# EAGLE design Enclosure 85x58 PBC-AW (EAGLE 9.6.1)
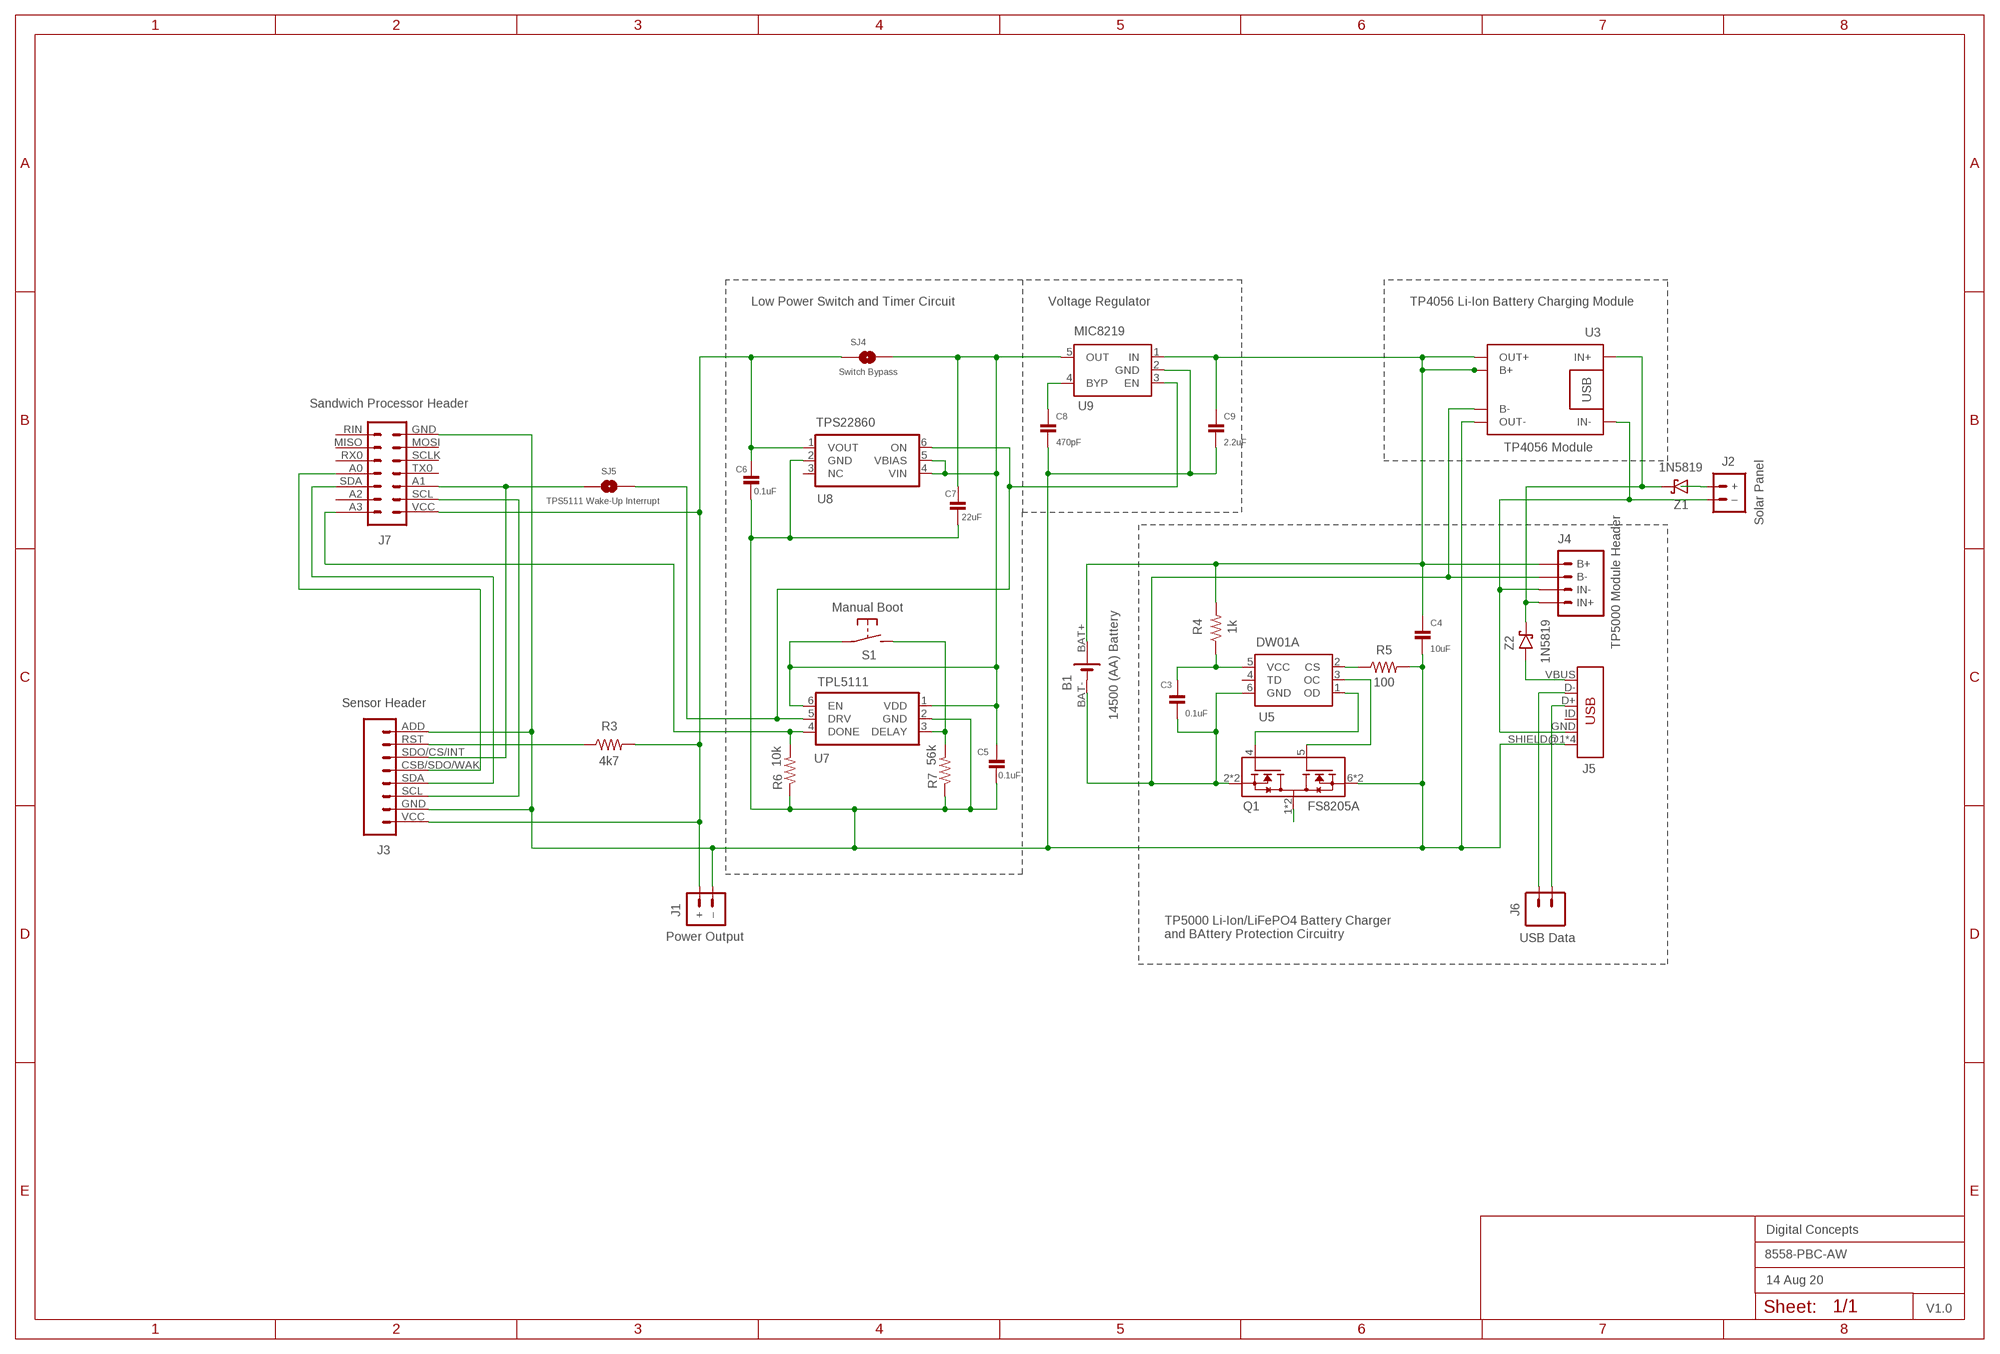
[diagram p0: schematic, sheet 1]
FRAME2 (A3L-LOC): DATE: 14 Aug 20; OWNER: Digital Concepts; TITLE: 8558-PBC-AW; VERSION: V1.0

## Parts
B1  14500 (AA) Battery  BATTERY-HOLDER-14500(AA)  [BATTERY-14500]
C3  0.1uF  CAPACITOR  [C0805]
C4  10uF  CAPACITOR  [C0805]
C5  0.1uF  CAPACITOR  [C0805]
C6  0.1uF  CAPACITOR  [C0805]
C7  22uF  CAPACITOR  [C0805]
C8  470pF  CAPACITOR  [C0805]
C9  2.2uF  CAPACITOR  [C0805]
J1  Power Output  JST-PH1.25-MALE  [JST-PH1.25]
J2  Solar Panel  JST-PH2.0-MALE  [JST-PH2.0]
J3  Sensor Header  HEADER-1X8-SENSOR  [CONN_08-SENSOR]
J4  TP5000 Module Header  TP5000-MODULE  [CONN_04-GENERIC]
J5  USB  USB_MINI-B_SMT  [USB-MINIB]
J6  USB Data  1X2-PIN-HEADER  [CONN_02-GENERIC]
J7  Sandwich Processor Header  HEADER-2X7-SANDWICH-PROCESSOR  [CONN_2X7-WIJNAND-PROCESSOR]
Q1  FS8205A  [SOP65P640X120-8N]
R3  4k7  RESISTORR0805  [R0805]
R4  1k  RESISTORR0805  [R0805]
R5  100  RESISTORR0805  [R0805]
R6  10k  RESISTORR0805  [R0805]
R7  56k  RESISTORR0805  [R0805]
S1  Manual Boot  MOMENTARY-SWITCH-2-PIN  [SWITCH-2-PAD]
SJ4  Switch Bypass  SJ  [SJ]
SJ5  TPS5111 Wake-Up Interrupt  SJ  [SJ]
U3  TP4056 Module  BATTERY-CHARGER-LI-PROT  [BATTERY-CHARGER-LI-PROT]
U5  DW01A  [SOT23-6]
U7  TPL5111  TPL5111DDCR  [SOT-23-6]
U8  TPS22860  [SOT-23-6]
U9  MIC8219  MIC5219XX  [SOT-23-5]
Z1  1N5819  1N5819-SOD-123  [SOD-123]
Z2  1N5819  1N5819-SOD-123  [SOD-123]

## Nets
GND: C4.2 C5.2 C6.2 C7.2 C8.2 C9.2 J1.-(–) J3.ADD J3.GND J5.SHIELD@1(SHIELD) J5.SHIELD@2(SHIELD) J5.SHIELD@3(SHIELD) J5.SHIELD@4(SHIELD) J7.GND Q1.6(S2) Q1.7(S2) R5.2 R6.1 R7.1 U3.OUT- U7.2(GND) U8.2(GND) U9.2(GND)
N$1: J2.+ Z1.A
N$2: J2.-(–) J4.2(IN-) J5.GND U3.IN-
N$3: R5.1 U5.2(CS)
N$4: Q1.1(D12) Q1.8(D12)
N$5: J4.1(IN+) U3.IN+ Z1.C Z2.C
N$6: B1.BAT+ C4.1 C9.1 J4.4(B+) R4.2 U3.B+ U3.OUT+ U9.1(IN)
N$7: C8.1 U9.4(BYP)
N$8: J3.SCL J7.SCL
N$9: J3.RST R3.1
N$10: J3.CSB/SDO/WAK J7.A0
N$11: J3.SDA J7.SDA
N$18: Q1.5(G2) U5.3(OC)
N$19: J5.VBUS Z2.A
N$20: Q1.4(G1) U5.1(OD)
N$21: J5.D+ J6.2
N$22: C3.1 R4.1 U5.5(VCC)
N$23: B1.BAT- C3.2 J4.3(B-) Q1.2(S1) Q1.3(S1) U3.B- U5.6(GND)
N$24: J5.D- J6.1
N$25: R7.2 S1.P$2(S) U7.3(DELAY)
N$26: C5.1 C7.1 S1.P$1(P) SJ4.2 U7.1(VDD) U7.6(EN) U8.4(VIN) U8.5(VBIAS) U9.5(OUT)
N$28: SJ5.2 U7.5(DRV) U8.6(ON) U9.3(EN)
N$29: J7.A3 R6.2 U7.4(DONE)
N$30: J3.SDO/CS/INT J7.A1 SJ5.1
VCC: C6.1 J1.+ J3.VCC J7.VCC R3.2 SJ4.1 U8.1(VOUT)
Unconnected: J5.ID J7.A2 J7.MISO J7.MOSI J7.RIN J7.RX0 J7.SCLK J7.TX0 U5.4(TD) U8.3(NC)

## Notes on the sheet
- Low Power Switch and Timer Circuit | Voltage Regulator | TP4056 Li-Ion Battery Charging Module
- TP5000 Li-Ion/LiFePO4 Battery Charger
  and BAttery Protection Circuitry

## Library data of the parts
B1 = digitalconcepts:BATTERY-HOLDER-14500(AA): 14500 (AA) battery holder
C3-C9 = digitalconcepts:CAPACITOR: 0805 Capacitor
J1 = digitalconcepts:JST-PH1.25-MALE: PH1.25 Male PCB Connector
J2 = digitalconcepts:JST-PH2.0-MALE: PH2.0 Male PCB Connector
J3 = digitalconcepts:HEADER-1X8-SENSOR: IoT Sensors 1x8 Pin Header for 'Sandwich' IoT Sensors
J4 = digitalconcepts:TP5000-MODULE: TP5000 Module Pin Header
J5 = digitalconcepts:USB_MINI-B: USB Mini-B Connector Breaks out 5 pins, and includes shield pins if needed.
J6 = digitalconcepts:1X2-PIN-HEADER: Single Row 2-Pin Header
J7 = digitalconcepts:HEADER-2X7-SANDWICH-PROCESSOR: 'Sandwixh' Processor 2x7 Pin Header for 'Sandwich' Processor/RFM95W PCBs
Q1 = FS8205A:FS8205A: N/A; AVAILABILITY: Unavailable; MF: Fortune Semiconductor; MP: FS8205A; PACKAGE: Package; PRICE: None
R3-R7 = digitalconcepts:RESISTOR: RESISTOR, American symbol; SPICEPREFIX: R
S1 = digitalconcepts:MOMENTARY-SWITCH-2-PIN: 2 Pin Momentary Switch
SJ4 SJ5 = digitalconcepts:SJ: Solder Jumper
U3 = digitalconcepts:BATTERY-CHARGER-LI-PROT: TP4056 Li Battery Charger module with PCB (rather than module) footprint
U5 = DW01A:DW01A; AVAILABILITY: Unavailable; DESCRIPTION: One Cell Lithium-ion/Polymer Battery Protection IC; MF: Fortune Semiconductor; MP: DW01A; PACKAGE: SOT-23-6 Fortune Semiconductor; PRICE: None
U7 = TPL5111DDCR:TPL5111DDCR: TPL5111 Nano-Power System Timer
U8 = TPL5111DDCR:TPS22860: Texas Instruments TPS22860 Ultra-Low Leakage Load Switch
U9 = digitalconcepts:MIC5219XX: VOLTAGE REGULATOR; OC_FARNELL: unknown; OC_NEWARK: unknown
Z1 Z2 = digitalconcepts:1N5819-SOD-123: 1N5819 Schottky Diode SOD-123

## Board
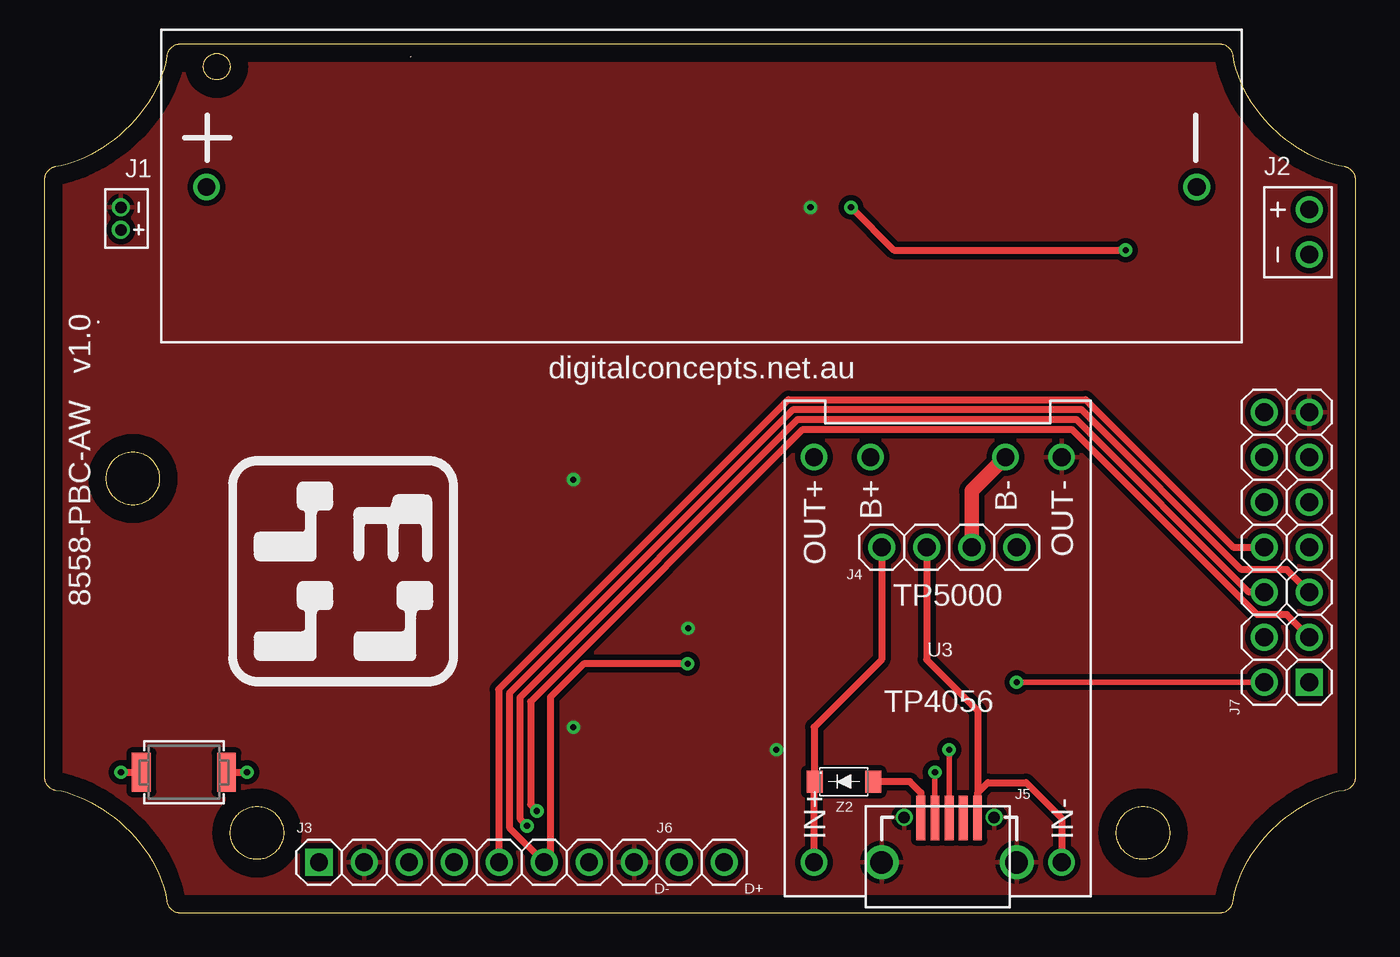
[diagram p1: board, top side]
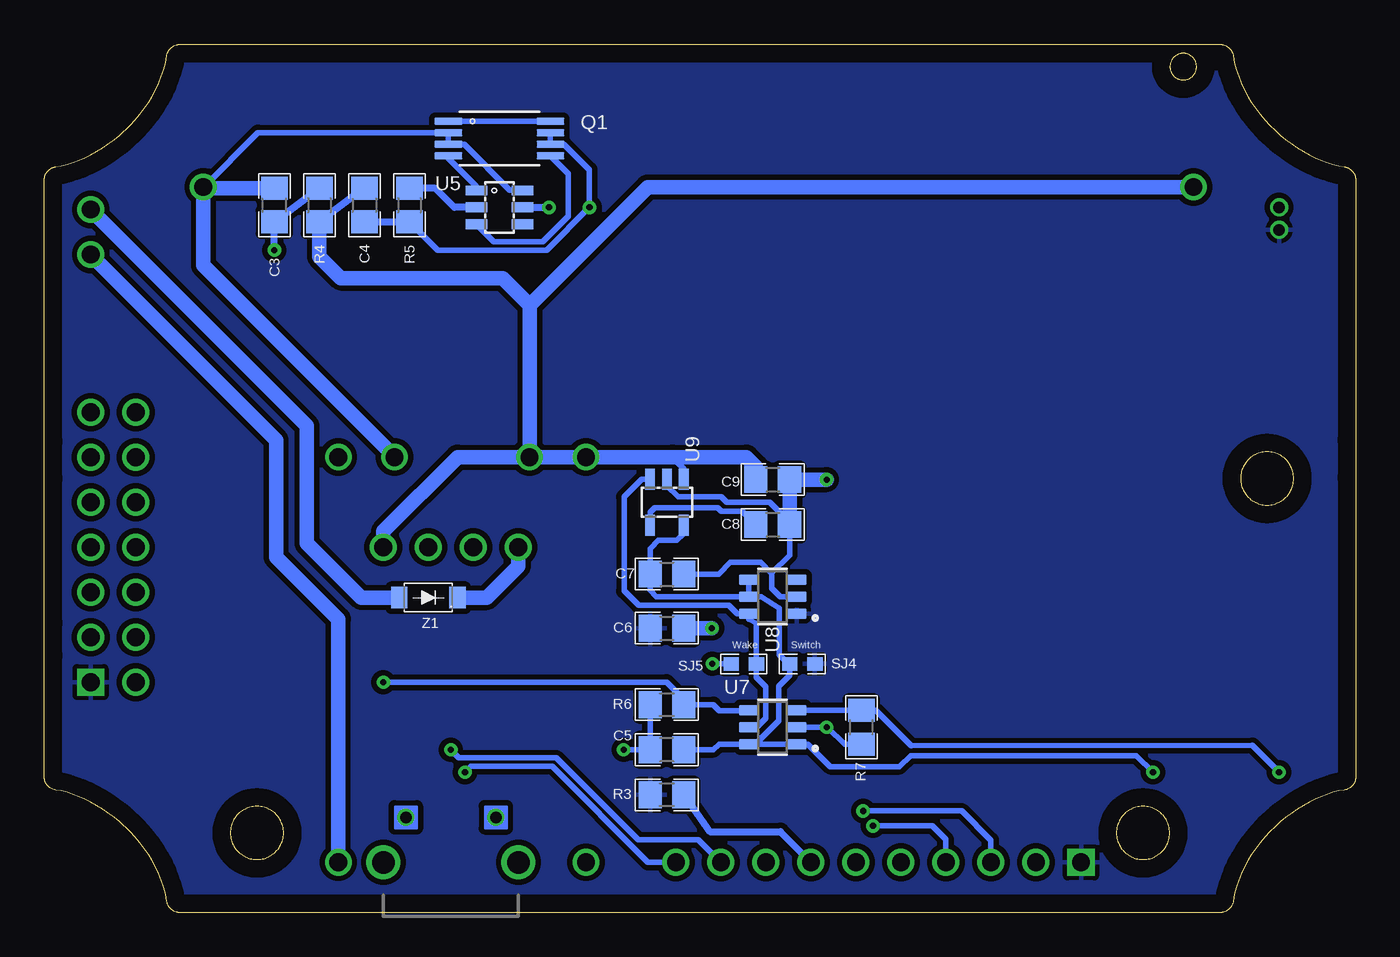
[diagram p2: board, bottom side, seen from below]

Size 74 x 49 mm. Coordinates in mm from the lower left corner, seen from the top.
Outline: 638 segments
Copper layers (1*16): Top 0.035mm / dielectric 1.5mm / Bottom 0.035mm
Design rules "default *": minimum track width 6mil, minimum drill 0.35mm, track to track 6mil, track to pad 6mil, pad to pad 6mil, via to via 6mil, smd to smd 6mil, copper to edge 40mil, drill to drill 6mil, minimum pad ring 1mil, minimum via ring 8mil, stop-mask expansion 4mil, vias tented up to drill 0mil, thermal gap 10mil

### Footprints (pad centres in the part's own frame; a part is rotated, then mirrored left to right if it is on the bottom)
BATTERY-14500 = drill 1: BAT+ -27.94,0; BAT- 27.94,0
C0805 = smd 1.3 x 1.5: 1 -0.95,0; 2 0.95,0
JST-PH1.25 = drill 0.65 pad 1.016: + -0.635,0; - 0.635,0
JST-PH2.0 = drill 1: + -1.27,0; - 1.27,0
CONN_08-SENSOR = drill 1 pad 1.524: ADD 17.78,0; CSB/SDO/WAK 10.16,0; GND 2.54,0; RST 15.24,0; SCL 5.08,0; SDA 7.62,0; SDO/CS/INT 12.7,0 | drill 1 pad 1.524 square: VCC 0,0
CONN_04-GENERIC = drill 1 pad 1.524: 1 0,0; 2 2.54,0; 3 5.08,0; 4 7.62,0
USB-MINIB = smd 2.5 x 0.5: D+ 2.5,0; D- 2.5,0.8; GND 2.5,-1.6; ID 2.5,-0.8; VBUS 2.5,1.6 | drill 1.27: SHIELD@1 0,3.81; SHIELD@2 0,-3.81 | drill 0.65 pad 0.762: SHIELD@3 2.54,2.54; SHIELD@4 2.54,-2.54
CONN_02-GENERIC = drill 1 pad 1.524: 1 0,0; 2 2.54,0
CONN_2X7-WIJNAND-PROCESSOR = drill 1 pad 1.524: A0 7.62,2.54; A1 5.08,0; A2 2.54,2.54; A3 0,2.54; GND 15.24,0; MISO 12.7,2.54; MOSI 12.7,0; RIN 15.24,2.54; RX0 10.16,2.54; SCL 2.54,0; SCLK 10.16,0; SDA 5.08,2.54; TX0 7.62,0 | drill 1 pad 1.524 square: VCC 0,0
SOP65P640X120-8N = smd 1.56 x 0.4: 1 -2.88,0.975; 2 -2.88,0.325; 3 -2.88,-0.325; 4 -2.88,-0.975; 5 2.88,-0.975; 6 2.88,-0.325; 7 2.88,0.325; 8 2.88,0.975
R0805 = smd 1.3 x 1.5: 1 -0.95,0; 2 0.95,0
SWITCH-2-PAD = smd 1.067 x 2.184: P$1 -2.4,0; P$2 2.4,0
SJ = smd 0.864 x 0.762: 1 -0.711,0; 2 0.711,0
BATTERY-CHARGER-LI-PROT = drill 1: B+ 10.795,3.81; B- 10.795,-3.81; IN+ -12.065,6.985; IN- -12.065,-6.985; OUT+ 10.795,6.985; OUT- 10.795,-6.985
SOT23-6 = smd 0.55 x 1.2: 1 -0.95,-1.3; 2 0,-1.3; 3 0.95,-1.3; 4 0.95,1.3; 5 0,1.3; 6 -0.95,1.3
SOT-23-6 = smd 1.1 x 0.6: 1 -1.35,0.95; 2 -1.35,0; 3 -1.35,-0.95; 4 1.35,-0.95; 5 1.35,0; 6 1.35,0.95
SOT-23-5 = smd 0.55 x 1.2: 1 -0.95,-1.3; 2 0,-1.3; 3 0.95,-1.3; 4 0.95,1.3; 5 -0.95,1.3
SOD-123 = smd 0.91 x 1.22: A -1.65,0; C 1.65,0

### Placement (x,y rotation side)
B1  37.09,40.94 0 top
C3  61.02,39.93 90 bottom
C4  55.94,39.93 270 bottom
C5  38.87,9.19 180 bottom
C6  38.87,16.05 0 bottom
C7  38.87,19.1 0 bottom
C8  32.9,21.89 0 bottom
C9  32.9,24.43 0 bottom
J1  4.32,39.16 90 top
J2  71.38,38.4 270 top
J3  15.5,2.84 0 top
J4  47.25,20.62 0 top
J5  51.06,2.84 90 top
J6  38.36,2.84 180 top
J7  71.38,13 90 top
Q1  48.32,43.69 0 bottom
R3  38.87,6.65 180 bottom
R4  58.48,39.93 270 bottom
R5  53.4,39.93 270 bottom
R6  38.87,11.73 0 bottom
R7  27.9,10.46 90 bottom
S1  7.88,7.92 180 top
SJ4  31.22,14.04 180 bottom
SJ5  34.53,14.04 0 bottom
U3  50.43,14.91 90 top
U5  48.32,39.8 270 bottom
U7  32.9,10.46 180 bottom
U8  32.9,17.83 180 bottom
U9  38.87,23.16 180 bottom
Z1  52.33,17.78 0 bottom
Z2  45.12,7.39 180 top

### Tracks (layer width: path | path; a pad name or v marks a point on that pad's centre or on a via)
GND  (via drill 0.35)
  Bottom 0.305: R6.1 C5.2 v41.31,9.19 | R5.2 51.81,37.39 45.65,37.39 v43.24,39.8 43.24,41.92 44.68,43.36 Q1.6 Q1.7 | U7.2 v29.85,10.46 29.83,10.48 v29.85,10.46 29.81,10.46 28.84,9.51 R7.1 | U8.2 32.47,17.83 32.95,18.31 32.95,19.12 32.98,19.15 | 32.98,19.15 33.59,19.76 35.29,19.76 35.95,19.1 C7.2 | 32.98,19.15 31.95,20.18 C8.2 31.95,22.03 33.08,23.16 35.49,23.16 35.8,23.47 38.23,23.47 38.87,24.1 U9.2
  Bottom 0.406: C4.2 R5.2
  Bottom 0.813: C8.2 C9.2 v29.85,24.43 | v36.33,16.05 C6.2
  pour Top (isolate 0.305): -1.44,50.36 -1.44,-1.54 75.56,-1.54 75.56,50.36
N$1
  Bottom 0.813: J2.+ 59.18,27.47 59.18,20.84 56.11,17.78 Z1.A
N$2
  Top 0.406: J4.2 49.79,14.27 52.66,11.4 J5.GND 52.66,6.75 53.25,7.34 55.4,7.34 57.41,5.33 U3.IN-
  Bottom 0.813: U3.IN- 57.41,16.56 60.92,20.06 60.92,26.67 J2.-
N$3
  Bottom 0.406: U5.2 50.86,39.8 51.94,40.88 R5.1
N$4
  Bottom 0.305: Q1.8 Q1.1
N$5
  Top 0.305: 43.44,7.36 Z2.C
  Top 0.406: U3.IN+ 43.44,7.36 | Z2.C 43.44,7.41 43.44,10.46 47.25,14.27 J4.1
  Bottom 0.813: J4.1 47.25,19.56 49.03,17.78 Z1.C
N$6
  Bottom 0.305: U9.1 37.92,25.06 38.56,25.7
  Bottom 0.406: C4.1 R4.2
  Bottom 0.813: U3.B+ U3.OUT+ 38.56,25.7 34.38,25.7 33.85,25.17 C9.1 | B1.BAT+ 39.96,40.94 46.62,34.29 | 46.62,34.29 U3.B+ | U3.B+ 50.68,25.7 54.87,21.51 J4.4 | R4.2 58.48,37.02 57.26,35.8 48.13,35.8 46.62,34.29
N$7
  Bottom 0.305: C8.1 34.61,22.65 35.81,22.65 36.01,22.86 39.55,22.86 39.82,22.59 U9.4
N$8  (via drill 0.35)
  Top 0.406: v27.79,5.74 27.44,6.09 27.44,11.91 42.81,27.28 57.97,27.28 68.43,16.81 70.11,16.81 J7.SCL
  Bottom 0.305: v27.79,5.74 22.23,5.74 20.58,4.09 J3.SCL
N$9
  Bottom 0.406: J3.RST 32.47,4.57 36.45,4.57 R3.1
N$10
  Top 0.406: J3.CSB/SDO/WAK 25.64,2.87 25.64,12.6 41.99,28.95 58.76,28.95 67.09,20.62 J7.A0
N$11  (via drill 0.35)
  Top 0.406: J7.SDA 67.98,18.08 58.22,27.84 42.53,27.84 26.83,12.14 26.83,5.31 v27.24,4.9
  Bottom 0.305: v27.24,4.9 23.88,4.9 23.12,4.14 J3.SDA
N$18
  Bottom 0.305: Q1.5 44.42,41.69 44.42,39.3 45.86,37.86 48.63,37.86 U5.3
N$19
  Top 0.406: Z2.A 48.85,7.39 49.46,6.78 J5.VBUS
N$20
  Bottom 0.305: Q1.4 51.2,42.56 49.62,40.98 U5.1
N$21  (via drill 0.35)
  Top 0.305: J5.D+ v51.06,9.19
  Bottom 0.305: v51.06,9.19 50.6,8.74 45.12,8.74 40.49,4.11 37.09,4.11 J6.2
N$22  (via drill 0.35)
  Top 0.406: v45.52,39.8 47.94,37.39 v61.02,37.39
  Bottom 0.406: R4.1 C3.1 v61.02,37.39 | U5.5 v45.52,39.8
N$23
  Top 0.813: U3.B- 52.33,23.8 J4.3
  Bottom 0.305: U5.6 47.04,40.77 47.73,40.77 50.31,43.36 Q1.3 Q1.2 61.95,44.01 65.01,40.94 B1.BAT- | U3.B- 54.24,25.73
  Bottom 0.813: 54.24,25.73 65.03,36.52 B1.BAT- 64.96,40.88 C3.2
N$24  (via drill 0.35)
  Top 0.305: J5.D- v50.26,7.92
  Bottom 0.305: v50.26,7.92 49.93,8.25 45.35,8.25 39.94,2.84 J6.1
N$25  (via drill 0.35)
  Top 0.406: v4.32,7.92 S1.P$2
  Bottom 0.305: v4.32,7.92 5.84,9.43 25.08,9.41 27.08,11.41 R7.2 U7.3
N$26  (via drill 0.35)
  Top 0.406: S1.P$1 v11.44,7.92
  Bottom 0.305: v11.44,7.92 12.38,8.86 25.12,8.86 25.75,8.24 29.64,8.24 30.91,9.51 U7.1 U7.6 | U8.5 33.55,17.83 32.52,17.17 32.52,14.55 32.01,14.04 SJ4.2 31.93,13.41 32.57,12.77 32.57,10.83 33.86,9.54 U7.6 | U8.5 U8.4 | C5.1 36.25,9.19 35.93,9.51 U7.6 | U8.5 39.46,17.83 39.82,18.18 C7.1 39.82,20.54 39.35,21 38.31,21 37.92,21.39 U9.5
N$28
  Bottom 0.305: U7.5 33.76,10.49 33.28,10.97 33.28,12.75 33.81,13.28 SJ5.2 33.81,16.34 34.25,16.56 U8.6 34.91,16.88 35.38,17.35 40.47,17.35 41.28,18.16 41.28,23.46 40.28,24.46 U9.3
N$29  (via drill 0.35)
  Top 0.305: J7.A3 v54.87,13
  Bottom 0.305: U7.4 34.28,11.39 35.9,11.39 36.25,11.73 R6.2 37.92,12.04 38.88,13 v54.87,13
N$30  (via drill 0.35)
  Top 0.406: J7.A1 70.11,19.35 67.55,19.35 58.5,28.39 42.27,28.39 26.24,12.37 26.24,4.8 J3.SDO/CS/INT 28.45,2.84 28.56,2.94 28.56,12.16 30.44,14.04 v36.3,14.04
  Bottom 0.305: SJ5.1 v36.3,14.04
VCC
  pour Bottom (isolate 0.305): -0.44,49.36 -0.44,-0.54 74.56,-0.54 74.56,49.36

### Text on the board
tPlace: J2 | J1 | digitalconcepts.net.au | 8558-PBC-AW v1.0 | TP5000 | TP4056 | D- | D+
bPlace: Switch | Wake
